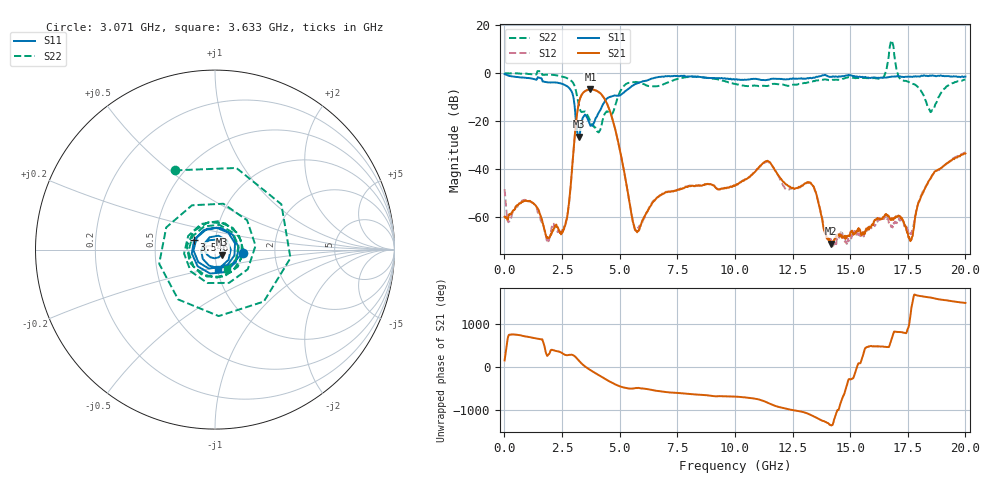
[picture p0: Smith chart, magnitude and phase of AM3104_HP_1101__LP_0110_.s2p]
!Created with skrf (http://scikit-rf.org).
# Hz S RI R 50.0
!freq ReS11 ImS11 ReS21 ImS21 ReS12 ImS12 ReS22 ImS22
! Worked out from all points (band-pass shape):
!   1601 points, 10 MHz to 20 GHz, reference 50 ohm
!   highest |S21| = -6.73 dB at 3.733 GHz (marker M1); lowest = -70.9 dB at 14.17 GHz (marker M2)
!   |S21| within 3 dB of the highest: 3.316 GHz to 4.281 GHz (965.2 MHz wide, 25.4 % of centre)
!   lowest |S11| = -26.5 dB at 3.221 GHz (marker M3), VSWR 1.10, Z = 53.9 - j2.97 ohm
!   |S11| at or under -10 dB: 2.994 GHz to 4.555 GHz (1.561 GHz wide, 41.4 % of centre)
!   |S22| runs from -24.7 to 13.6 dB; largest |S21 - S12| = 0.028
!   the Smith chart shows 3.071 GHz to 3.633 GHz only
!   S11 on the Smith chart (normalised r, x): 3.071 GHz: 1.36, -0.05; 3.546 GHz: 0.79, +0.09; 3.633 GHz: 1.01, -0.22
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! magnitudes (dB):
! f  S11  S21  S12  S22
! 10 MHz  -0.4  -59.8  -48.3  -0.1
! 209.9 MHz  -1.1  -59.1  -61.7  -0.1
! 1.034 GHz  -2.0  -53.2  -53.2  -0.4
! 1.872 GHz  -3.8  -68.7  -70.7  -0.7
! 2.546 GHz  -4.6  -65.3  -65.4  -1.5
! 3.071 GHz  -16.2  -24.1  -24.1  -6.1
! 3.221 GHz  -26.5  -12.9  -12.9  -12.9
! 3.346 GHz  -21.1  -9.1  -9.2  -16.2
! 3.546 GHz  -17.9  -7.2  -7.3  -16.5
! 3.633 GHz  -19.4  -6.9  -7.0  -18.0
! 3.733 GHz  -21.9  -6.7  -6.8  -20.3
! 4.62 GHz  -9.8  -16.9  -17.0  -17.0
! 5.707 GHz  -4.5  -65.6  -65.5  -3.7
! 6.682 GHz  -1.6  -51.5  -51.6  -5.4
! 10.01 GHz  -2.7  -46.9  -46.8  -4.5
! 11.39 GHz  -2.9  -36.6  -36.8  -5.3
! 13.34 GHz  -2.1  -46.4  -46.3  -3.5
! 14.17 GHz  -1.5  -70.9  -69.8  -2.9
! 16.68 GHz  -1.6  -59.7  -62.4  7.2
! 17.63 GHz  -1.5  -69.7  -66.7  -4.1
! 18.5 GHz  -1.1  -43.7  -43.7  -16.2
! 20 GHz  -1.4  -33.5  -33.0  -2.7
